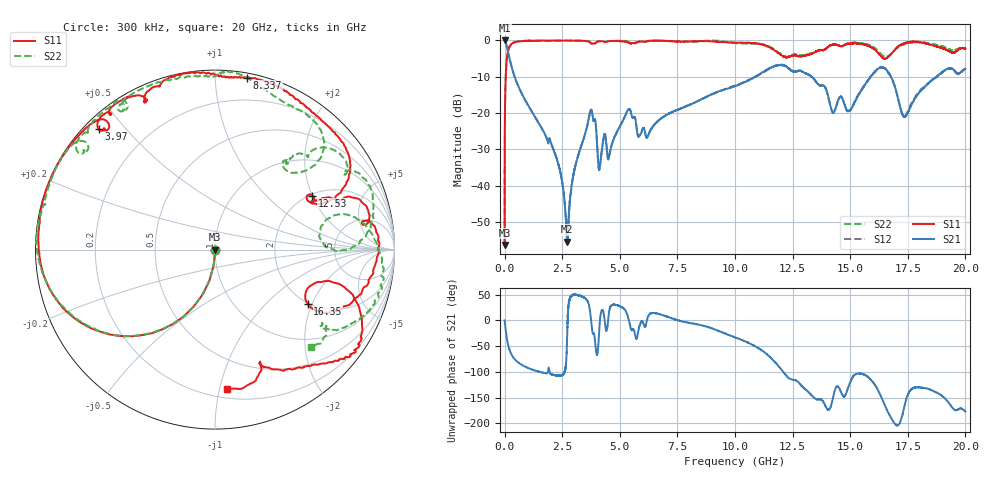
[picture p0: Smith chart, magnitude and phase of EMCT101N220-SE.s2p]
!EMCT101N220
!Johanson Technology Inc.
!www.johansontechnology.com
!Test Board Conditions:
!Substrate Type  RO4350B
!Substrate Thickness  10 mil
!Substrate Dk  3.66
!TL Type: GCPW
!TL Trace Width  22 mil
!TL Gap  14 mil
!PART MODE SINGLE ENDED (AKA BYPASS)
!DUT TOPOLOGY	SERIES-SHUNT
# MHz S  dB  R 50
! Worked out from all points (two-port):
!   20001 points, 300 kHz to 20 GHz, reference 50 ohm
!   highest |S21| = 0.00 dB at 2.3 MHz (marker M1); lowest = -55.4 dB at 2.718 GHz (marker M2)
!   |S21| within 3 dB of the highest: start of sweep to 142.9 MHz
!   lowest |S11| = -56.3 dB at 300 kHz (marker M3), VSWR 1.00, Z = 50.1 - j0.0814 ohm
!   |S11| at or under -10 dB: start of sweep to 48.47 MHz
!   |S22| runs from -56.7 to 0.0 dB; largest |S21 - S12| = 0.014
!   S11 on the Smith chart (normalised r, x): 300 kHz: 1.00, -0.00; 3.97 GHz: 0.04, +0.42; 8.337 GHz: 0.03, +1.20; 12.53 GHz: 2.05, +2.01; 16.35 GHz: 1.97, -1.86; 20 GHz: 0.27, -1.05
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0.3  -56.34 -32.2  -0.01 -0.2  -0.00 -0.2  -56.67 -40.0
2.3  -36.04 -87.7  -0.00 -1.0  -0.01 -1.0  -36.11 -87.9
105.298  -4.64 -127.3  -1.88 -37.0  -1.87 -37.0  -4.69 -127.3
237.296  -1.47 -150.6  -5.58 -60.0  -5.57 -60.1  -1.53 -150.6
2193.267  -0.02 158.3  -31.34 -106.5  -31.24 -106.7  -0.10 162.1
2718.259  -0.03 148.7  -55.40 -24.9  -55.14 -29.0  -0.05 155.5
3334.25  -0.11 137.6  -28.90 46.6  -28.93 46.4  -0.04 147.1
3729.244  -0.70 130.1  -19.22 9.7  -19.23 9.9  -0.64 140.3
3970.24  -0.62 134.0  -24.14 -60.5  -24.15 -60.6  -0.59 144.7
4129.238  -0.23 130.8  -35.06 -4.7  -35.07 -5.1  -0.20 141.2
5367.219  -0.59 114.9  -19.03 4.4  -19.05 4.8  -0.43 121.2
5842.212  -0.34 112.6  -26.31 -12.6  -26.22 -12.2  -0.36 123.7
6667.2  -0.06 98.1  -22.15 12.7  -22.13 12.4  -0.13 114.4
8337.175  -0.22 79.4  -16.88 -7.7  -16.81 -7.9  -0.27 89.4
10000.15  -0.60 50.1  -12.60 -33.0  -12.44 -33.1  -0.70 69.9
12532.11  -4.15 29.0  -8.56 -115.3  -8.51 -115.7  -3.94 51.7
13334.1  -3.68 25.5  -10.01 -146.0  -10.02 -146.1  -3.51 50.2
14939.08  -0.89 7.4  -19.45 -127.2  -19.36 -126.0  -0.77 26.9
16351.06  -4.45 -30.4  -7.38 -149.1  -7.54 -149.5  -3.87 0.6
16667.05  -4.45 -17.7  -8.90 179.7  -9.04 -179.4  -4.26 12.8
17363.04  -0.75 -26.8  -21.06 -164.9  -20.88 -162.7  -0.98 3.6
20000  -2.20 -85.3  -7.78 -177.2  -7.82 -175.4  -2.37 -45.3
